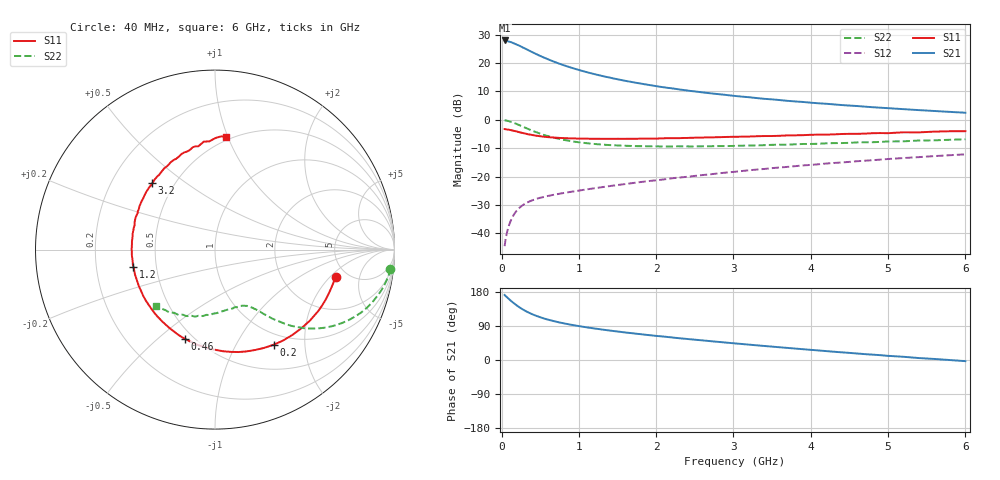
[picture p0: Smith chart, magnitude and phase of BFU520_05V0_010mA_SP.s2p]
! Filename:  P:\Prog\Test\Noise\ATS_data\Testdata_Net\03 Spar\BFU520_APG2013_37_A05_05p0V_010mA_SP_CM01_D.s2p
! Date/Time: Fri 26/Apr/2013 13:00:08
! BFU520_APG2013_37_A05_05p0V_1to20mA_SP_CM01_Bias6_R.s2p
! MDIF S-parameter v. bias file
! BFU520_APG2013_37_A05_05p0V_1to20mA_SP_CM01
! Date/time Tue Apr 23 15:26:19 2013
! VAR V_out= 5.0010
! VAR I_out= 9.9900
! VAR V_in= 0.8386
! VAR I_in= 0.1144
! Device data file deembeded for feedlines and parallel
! Original file: \03 Spar\BFU520_APG2013_37_A05_05p0V_010mA_SP_CM01_R.s2p
! Feed-files: PR047V01_250413_Feed1.s2p, PR047V01_250413_Feed2.s2p
! Parallel-file: PR047V01_250413_Par.s2p
# MHz S MA R 50
!  Freq-MHz  S11-mag  S11-arg  S21-mag  S21-arg  S12-mag  S12-arg  S22-mag  S22-arg
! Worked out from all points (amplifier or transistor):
!   98 points, 40 MHz to 6 GHz, reference 50 ohm
!   highest |S21| = 28.0 dB at 40 MHz (marker M1)
!   |S21| within 3 dB of that: start of sweep to 316.2 MHz
!   unconditionally stable (mu >= 1): 1.746 GHz to 3.84 GHz
!   at 300 MHz: K = 0.31, MSG = 27.4 dB, |S12| = -29.6 dB
!   at 1.6 GHz: K = 0.97, MSG = 18.2 dB, |S12| = -22.6 dB
!   at 6 GHz: K = 0.85, MSG = 7.3 dB, |S12| = -12.1 dB
!   S11 on the Smith chart (normalised r, x): 40 MHz: 4.04, -2.30; 200 MHz: 0.83, -1.44; 460 MHz: 0.45, -0.62; 1.2 GHz: 0.37, -0.09; 3.2 GHz: 0.38, +0.38; 6 GHz: 0.47, +0.99
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40  0.6883 -12.6  25.05 171.6  0.005974 84.2  0.9829 -6.2
50  0.685 -15.8  25.03 169.1  0.007489 82.9  0.9807 -7.7
60  0.6816 -18.6  24.59 167.7  0.008906 81.1  0.9746 -9.4
120  0.6603 -36.9  23.46 156.5  0.01688 73.4  0.9269 -18.1
160  0.6415 -48.0  22.28 149.8  0.02154 68.6  0.8872 -23.2
200  0.6227 -58.4  21.09 143.6  0.02552 64.6  0.8419 -27.8
240  0.6024 -68.2  19.93 137.9  0.02893 61.3  0.7981 -31.7
300  0.5765 -81.3  18.18 130.6  0.03317 57.2  0.7347 -36.5
380  0.5468 -96.2  16.01 122.4  0.03748 53.4  0.6599 -41.5
460  0.5245 -108.5  14.19 115.8  0.04102 51.0  0.5997 -45.1
550  0.5047 -120.5  12.51 109.5  0.04397 49.2  0.5421 -47.9
700  0.4862 -135.4  10.33 101.4  0.04864 48.1  0.478 -51.3
850  0.4758 -147.3  8.753 95.0  0.05283 48.1  0.4337 -53.7
1050  0.4669 -160.1  7.247 87.8  0.05827 48.8  0.3958 -56.4
1200  0.4647 -167.8  6.406 83.2  0.06244 49.5  0.3769 -58.3
1600  0.464 175.6  4.878 72.7  0.07419 51.2  0.3503 -63.4
2050  0.4719 161.9  3.832 62.7  0.08786 52.4  0.3409 -70.0
3100  0.5056 135.0  2.575 42.4  0.1253 52.0  0.3513 -87.1
3200  0.5089 133.4  2.507 40.6  0.1298 51.7  0.3541 -88.4
4100  0.5498 114.7  1.96 25.2  0.1655 47.8  0.3798 -104.1
5200  0.6051 95.9  1.545 8.5  0.2129 40.9  0.4193 -122.9
6000  0.6325 84.3  1.337 -3.0  0.2475 34.5  0.4561 -136.4
